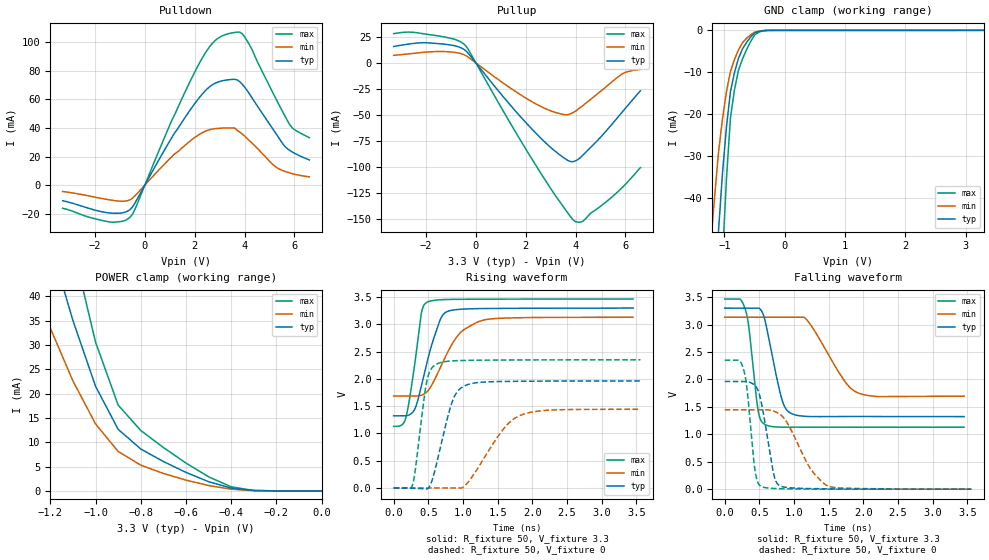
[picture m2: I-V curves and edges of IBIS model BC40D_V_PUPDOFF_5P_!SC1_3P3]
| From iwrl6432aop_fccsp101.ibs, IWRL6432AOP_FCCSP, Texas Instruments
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|   Model Cell BC40D_V_PUPDOFF_5P_!SC1_3P3
|BC40D_V_PUPDOFF_5P_!SC1_3P3
[Model]   BC40D_V_PUPDOFF_5P_!SC1_3P3
Model_type   I/O
Polarity   Non-Inverting
Enable   Active-Low
Vinl =  0.8V
Vinh =  2V
Cref =  15pF
Rref =  100.0000M
Vref =  0V
Vmeas =  1.65
C_comp   2.059994p   1.862014p   2.067327p
|[Input load] weak_pupdoff
|[Output drive] fast
|[supplytol] 5
|[temp] ind
[Model Spec]
Vinl   0.8V   0.8V   0.8V
Vinh   2V   2V   2V
[Temperature Range]   25   125   -40
[Voltage Range]   3.3   3.135   3.465
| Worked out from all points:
|   slope of the pulldown table from 0 to 0.495 V, typ, clamps not added: 31.8 ohm
|   slope of the pullup table from 0 to 0.495 V, typ, clamps not added: 33.3 ohm
|   GND clamp passes 1 mA (typ) near -0.53 V on its own axis
|   POWER clamp passes 1 mA (typ) near -0.43 V on its own axis
|   rising waveform, R_fixture 50, V_fixture 3.3: 20-80 % time 251ps typ, 371ps min, 151ps max; typ from 1.32 V to 3.3 V
|   rising waveform, R_fixture 50, V_fixture 0: 20-80 % time 232ps typ, 456ps min, 141ps max; typ from 0 V to 1.96 V
|   falling waveform, R_fixture 50, V_fixture 3.3: 20-80 % time 196ps typ, 407ps min, 120ps max; typ from 3.3 V to 1.32 V
|   falling waveform, R_fixture 50, V_fixture 0: 20-80 % time 159ps typ, 360ps min, 107ps max; typ from 1.96 V to 0 V
| Nom Voltages:
|   VDD=1.1, VDDS=3.3, VDDS18=1.8, ESD_BIASFET=0, VSS=0, VSSS=0
| Min Voltages:
|   VDD=1.045, VDDS=3.135, VDDS18=1.71, ESD_BIASFET=0, VSS=0, VSSS=0
| Max Voltages:
|   VDD=1.16, VDDS=3.465, VDDS18=1.89, ESD_BIASFET=0, VSS=0, VSSS=0
[POWER_clamp]
|   voltage   I(typ)   I(min)   I(max)
-3.3V     446.9mA    437.1mA    604mA
-1.267V   62.17mA    41.49mA    88.04mA
-1.233V   56.52mA    37.49mA    80.24mA
-1.133V   40.34mA    26.26mA    57.63mA
-1.067V   30.56mA    19.69mA    43.69mA
-1.033V   26.05mA    16.74mA    37.16mA
-1V       21.55mA    13.79mA    30.63mA
-900mV    12.68mA    8.13mA     17.66mA
-800mV    8.63mA     5.305mA    12.44mA
-600mV    3.813mA    2.231mA    5.735mA
-400mV    580.7uA    357.4uA    841.8uA
0V        4.589uA    2.331uA    8.159uA
[Pulldown]
|   voltage   I(typ)   I(min)   I(max)
-3.3V     -10.92mA   -4.469mA   -16.24mA
-1.4V     -19.52mA   -10.37mA   -25.81mA
-600mV    -17.22mA   -10.34mA   -22.6mA
-400mV    -12.67mA   -7.623mA   -17.05mA
1.2V      36.7mA     21.92mA    49.35mA
2.1V      59.3mA     34.49mA    82.4mA
2.7V      70.09mA    39.15mA    99.03mA
3.3V      73.56mA    39.95mA    105.7mA
3.9V      70.66mA    35.84mA    106mA
5.2V      37.64mA    13.39mA    62.46mA
5.8V      24.43mA    8.578mA    42.66mA
6.6V      17.6mA     5.765mA    33.17mA
[Pullup]
|   voltage   I(typ)   I(min)   I(max)
-3.3V     15.77mA    7.22mA     28.03mA
-2.7V     18.05mA    8.673mA    29.54mA
-1.9V     19.23mA    10.53mA    27.2mA
-900mV    16.69mA    10.25mA    22.94mA
-400mV    11.53mA    6.969mA    16.15mA
1.4V      -40.96mA   -24.37mA   -58.54mA
2.6V      -72.01mA   -41.71mA   -105.6mA
3.6V      -92.16mA   -49.74mA   -141mA
4V        -93.88mA   -46.2mA    -152.2mA
4.3V      -88.33mA   -40.72mA   -151.7mA
5.9V      -46.29mA   -10.2mA    -118.8mA
6.6V      -26.71mA   -6.269mA   -100.4mA
[GND_clamp]
|   voltage   I(typ)   I(min)   I(max)
-3.3V     -787.2mA   -627.7mA   -1.235A
-1.233V   -85.66mA   -52.14mA   -138.8mA
-1.167V   -66.47mA   -40.37mA   -107.7mA
-1.1V     -48.25mA   -29.37mA   -77.98mA
-1.033V   -34.27mA   -21.19mA   -54.56mA
-966.7mV  -23.06mA   -14.66mA   -35.5mA
-900mV    -14.61mA   -9.789mA   -20.83mA
-833.3mV  -10.05mA   -6.934mA   -14.15mA
-700mV    -4.416mA   -2.931mA   -6.81mA
-500mV    -621.6uA   -443.6uA   -1.094mA
-300mV    -17.13uA   -24.35uA   -23.51uA
3.3V      4.589uA    5.188uA    6.318uA
[Ramp]
| variable   typ   min   max
dV/dt_f  1.1959432/0.19778326n 0.88997478/0.42010629n  1.4076426/0.12045204n
dV/dt_r  1.1917501/0.23458044n 0.88925157/0.46804062n  1.4206668/0.14157829n
R_load = 50
[Rising Waveform]
R_fixture = 50
V_fixture = 3.3
V_fixture_min = 3.135
V_fixture_max = 3.465
|   time   V(typ)   V(min)   V(max)
0s        1.323V     1.687V     1.129V
178.2ps   1.324V     1.687V     1.297V
304.7ps   1.446V     1.687V     2.276V
398.7ps   1.871V     1.7V       3.195V
481.7ps   2.309V     1.765V     3.406V
653.8ps   3.025V     2.155V     3.45V
722.6ps   3.193V     2.343V     3.455V
946.6ps   3.276V     2.827V     3.46V
1.239ns   3.29V      3.057V     3.463V
3.453ns   3.299V     3.131V     3.465V
[Rising Waveform]
R_fixture = 50
V_fixture = 0
V_fixture_min = 0
V_fixture_max = 0
|   time   V(typ)   V(min)   V(max)
0s        0V         0V         0V
272.8ps   -6.681mV   0V         57.86mV
474.8ps   -20.71mV   0V         1.934V
537.3ps   78.73mV    0V         2.176V
615.7ps   426mV      0V         2.269V
850ps     1.601V     0V         2.331V
1.042ns   1.884V     59.9mV     2.34V
1.571ns   1.953V     1.06V      2.347V
1.827ns   1.957V     1.332V     2.348V
3.559ns   1.963V     1.443V     2.351V
[Falling Waveform]
R_fixture = 50
V_fixture = 3.3
V_fixture_min = 3.135
V_fixture_max = 3.465
|   time   V(typ)   V(min)   V(max)
0s        3.299V     3.134V     3.464V
297.1ps   3.299V     3.134V     3.277V
347.5ps   3.299V     3.134V     2.96V
479.2ps   3.299V     3.134V     1.457V
581.1ps   3.075V     3.134V     1.179V
822.1ps   1.65V      3.134V     1.13V
962ps     1.378V     3.134V     1.13V
1.186ns   1.326V     3.084V     1.13V
1.91ns    1.326V     1.762V     1.129V
3.453ns   1.322V     1.695V     1.129V
[Falling Waveform]
R_fixture = 50
V_fixture = 0
V_fixture_min = 0
V_fixture_max = 0
|   time   V(typ)   V(min)   V(max)
0s        1.963V     1.448V     2.35V
273.4ps   1.963V     1.448V     2.179V
326.7ps   1.958V     1.448V     1.774V
436.6ps   1.889V     1.448V     346mV
524.2ps   1.602V     1.448V     51.4mV
709.5ps   262.9mV    1.42V      13.06mV
807.3ps   55.33mV    1.355V     7.941mV
1.237ns   10.47mV    375.2mV    0V
1.49ns    6.801mV    58.45mV    0V
3.559ns   0V         3.299mV    0V
